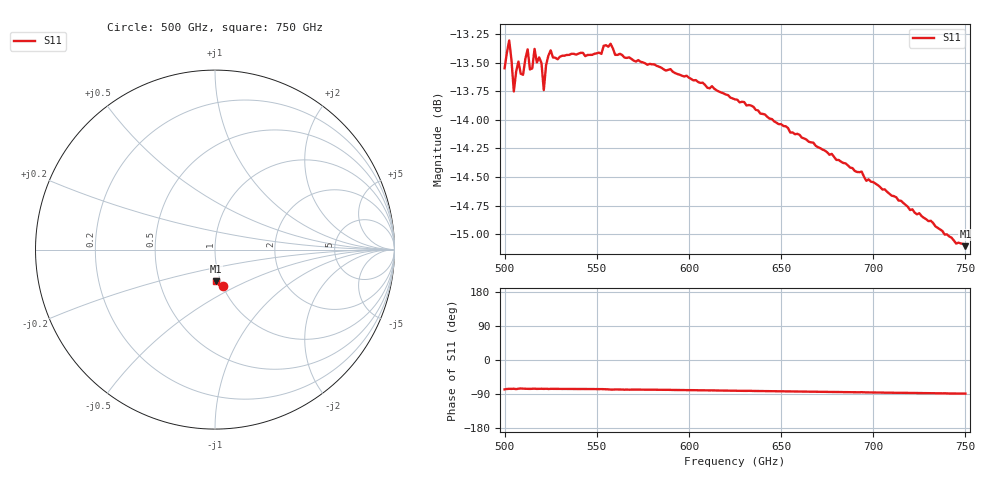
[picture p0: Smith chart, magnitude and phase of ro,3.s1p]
!Created with mwavepy.
!Created with skrf (http://scikit-rf.org).
# GHz S RI R 50.0
!freq ReS11 ImS11
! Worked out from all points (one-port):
!   201 points, 500 GHz to 750 GHz, reference 50 ohm
!   lowest |S11| = -15.1 dB at 750 GHz (marker M1), VSWR 1.43, Z = 47.4 - j17.2 ohm
!   |S11| at or under -10 dB: start of sweep to end of sweep
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500  0.0455 -0.2051
502.5  0.0521 -0.2097
505  0.0505 -0.199
506.25  0.0474 -0.204
507.5  0.0518 -0.2051
510  0.0518 -0.2022
512.5  0.0519 -0.2078
513.75  0.0497 -0.2039
515  0.0514 -0.2037
516.25  0.0534 -0.2075
517.5  0.05 -0.2053
520  0.0517 -0.2048
521.25  0.0488 -0.1997
522.5  0.0515 -0.2044
525  0.0515 -0.2077
526.25  0.0507 -0.2063
531.25  0.0503 -0.2068
552.5  0.0489 -0.2075
553.75  0.0484 -0.2094
557.5  0.0447 -0.2107
560  0.0455 -0.2081
562.5  0.045 -0.2084
593.75  0.0391 -0.2052
625  0.0318 -0.2012
656.25  0.0246 -0.1955
687.5  0.0159 -0.1895
718.75  0.0101 -0.1825
750  0.00392 -0.1757
